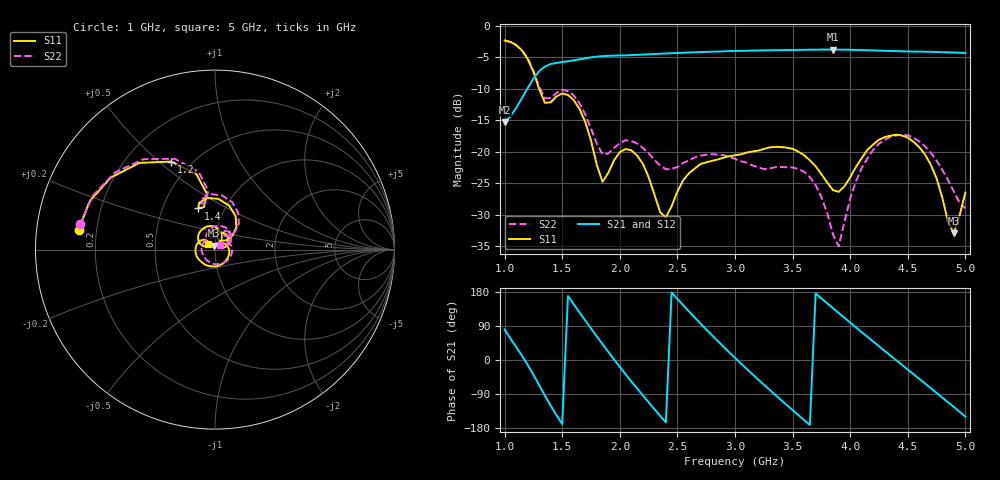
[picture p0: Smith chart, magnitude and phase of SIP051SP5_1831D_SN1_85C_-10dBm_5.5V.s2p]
# GHz  S  dB  R  50
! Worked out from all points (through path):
!   81 points, 1 GHz to 5 GHz, reference 50 ohm
!   highest |S21| = -3.74 dB at 3.85 GHz (marker M1); lowest = -15.3 dB at 1 GHz (marker M2)
!   lowest |S11| = -33.0 dB at 4.9 GHz (marker M3), VSWR 1.05, Z = 49.5 + j2.17 ohm
!   |S11| at or under -10 dB: 1.3 GHz to end of sweep
!   |S22| runs from -35.0 to -2.3 dB; largest |S21 - S12| = 0.0027
!   S11 on the Smith chart (normalised r, x): 1 GHz: 0.13, +0.07; 1.2 GHz: 0.39, +0.55; 1.4 GHz: 0.75, +0.37; 5 GHz: 0.93, +0.06
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1  -2.30 171.7  -15.34 80.8  -15.32 80.9  -2.33 169.4
1.2  -5.23 116.4  -9.89 -12.6  -9.87 -12.6  -5.14 113.9
1.4  -12.13 112.0  -6.05 -120.5  -6.05 -120.5  -11.44 106.9
1.55  -10.95 86.2  -5.61 168.9  -5.61 168.9  -10.34 82.2
1.7  -15.25 46.3  -5.13 104.4  -5.12 104.5  -14.07 47.7
1.85  -24.76 60.6  -4.79 41.8  -4.77 41.8  -20.38 52.3
2  -20.04 71.7  -4.68 -18.2  -4.66 -18.1  -18.62 62.1
2.2  -21.90 24.2  -4.54 -93.4  -4.54 -93.4  -19.38 33.6
2.35  -29.59 18.5  -4.41 -147.1  -4.39 -147.1  -22.18 27.5
2.5  -26.33 45.4  -4.29 161.4  -4.27 161.4  -22.41 31.0
2.7  -21.94 -2.4  -4.13 96.4  -4.13 96.5  -20.61 12.0
3  -20.54 -89.0  -3.97 5.8  -3.96 5.8  -21.12 -57.4
3.15  -19.95 -125.5  -3.91 -37.1  -3.90 -37.1  -22.16 -106.6
3.35  -19.22 -167.2  -3.85 -92.2  -3.85 -92.2  -22.44 177.4
3.7  -22.29 134.8  -3.77 175.6  -3.76 175.5  -25.32 81.2
3.85  -26.09 138.0  -3.74 136.9  -3.73 136.9  -33.10 78.3
3.9  -26.36 148.0  -3.75 124.2  -3.75 124.2  -35.00 113.9
4.1  -21.00 158.8  -3.83 73.5  -3.80 73.6  -22.57 134.3
4.35  -17.44 120.0  -3.97 11.6  -3.97 11.5  -17.64 87.3
4.65  -20.44 67.8  -4.09 -62.0  -4.09 -62.1  -19.14 33.9
4.9  -32.98 101.9  -4.21 -124.2  -4.20 -124.2  -26.32 20.8
5  -26.49 140.6  -4.29 -149.4  -4.29 -149.4  -29.01 41.6
